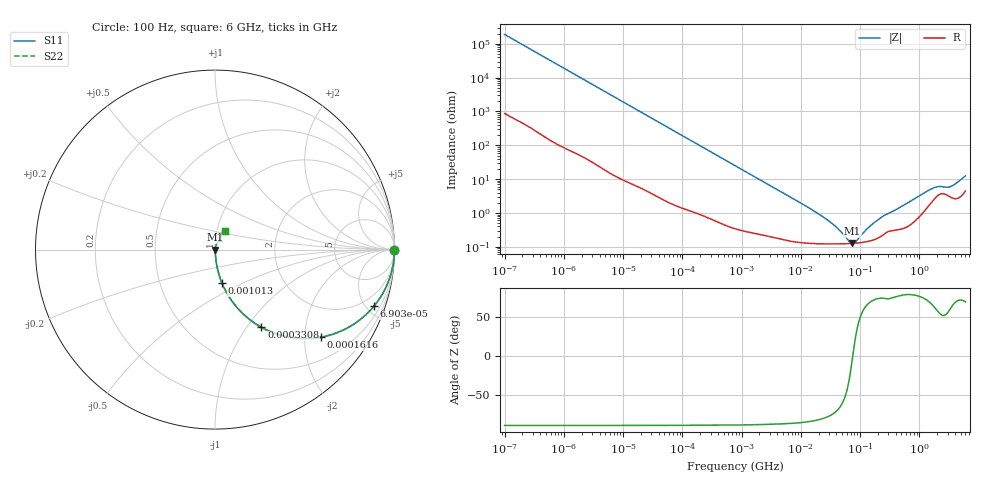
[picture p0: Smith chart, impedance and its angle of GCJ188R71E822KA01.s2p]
!Murata Part Number: GCJ188R71E822KA01
!These Parameters are Measured in Series Mode Connection
!Data Generated on Mar 13, 2026
!  o--ll--o
!Port1  Port2
!  o------o
!Operation Temp=25[degC], DC Bias Voltage=0[V]
!Freq. Start=100[Hz] Stop=6[GHz] 401[Steps]
# Hz S RI R 50
!Freq.(Hz) S11(Real) S11(Imag) S21(Real) S21(Imag) S12(Real) S12(Imag) S22(Real) S22(Imag)
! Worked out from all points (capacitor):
!   401 points, 100 Hz to 6 GHz, reference 50 ohm
!   read as one part in series: C = 8.4 nF near 109 Hz
!   lowest |Z| = 126 mohm at 74.56 MHz (marker M1)
!   series resonance near 75.5 MHz, so ESL is about 530 pH
!   S11 on the Smith chart (normalised r, x): 100 Hz: open; 69.03 kHz: 1.04, -5.59; 161.6 kHz: 1.02, -2.40; 330.8 kHz: 1.01, -1.18; 1.013 MHz: 1.01, -0.39; 6 GHz: 1.09, +0.23
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100  1 -0.000529  2.7e-06 0.000529  2.7e-06 0.000529  1 -0.000529
2008  0.9998 -0.0105  0.000163 0.0105  0.000163 0.0105  0.9998 -0.0105
12041  0.9958 -0.0625  0.00424 0.0625  0.00424 0.0625  0.9958 -0.0625
40335  0.9569 -0.2001  0.0431 0.2001  0.0431 0.2001  0.9569 -0.2001
69028  0.8849 -0.3159  0.1151 0.3159  0.1151 0.3159  0.8849 -0.3159
103284  0.776 -0.4133  0.224 0.4133  0.224 0.4133  0.776 -0.4133
161617  0.5885 -0.4878  0.4115 0.4878  0.4115 0.4878  0.5885 -0.4878
330837  0.2588 -0.4328  0.7412 0.4328  0.7412 0.4328  0.2588 -0.4328
774597  0.0625 -0.2354  0.9375 0.2354  0.9375 0.2354  0.0625 -0.2354
1013323  0.0385 -0.1849  0.9615 0.1849  0.9615 0.1849  0.0385 -0.1849
3103719  0.00595 -0.063  0.9941 0.063  0.9941 0.063  0.00595 -0.063
1.555665e7  0.0014 -0.0122  0.9986 0.0122  0.9986 0.0122  0.0014 -0.0122
3.482834e7  0.00124 -0.0045  0.9988 0.0045  0.9988 0.0045  0.00124 -0.0045
6.518806e7  0.00125 -0.000777  0.9988 0.000777  0.9988 0.000777  0.00125 -0.000777
7.455971e7  0.00126 -6.49e-05  0.9987 6.49e-05  0.9987 6.49e-05  0.00126 -6.49e-05
8.527865e7  0.00128 0.000646  0.9987 -0.000646  0.9987 -0.000646  0.00128 0.000646
1.669249e8  0.00161 0.00465  0.9984 -0.00465  0.9984 -0.00465  0.00161 0.00465
3.124326e8  0.00297 0.00953  0.997 -0.00953  0.997 -0.00953  0.00297 0.00953
1.565993e9  0.0213 0.0448  0.9787 -0.0448  0.9787 -0.0448  0.0213 0.0448
2.048624e9  0.0339 0.047  0.9661 -0.047  0.9661 -0.047  0.0339 0.047
3.352442e9  0.0311 0.0492  0.9689 -0.0492  0.9689 -0.0492  0.0311 0.0492
6e9  0.0545 0.1056  0.9455 -0.1056  0.9455 -0.1056  0.0545 0.1056
